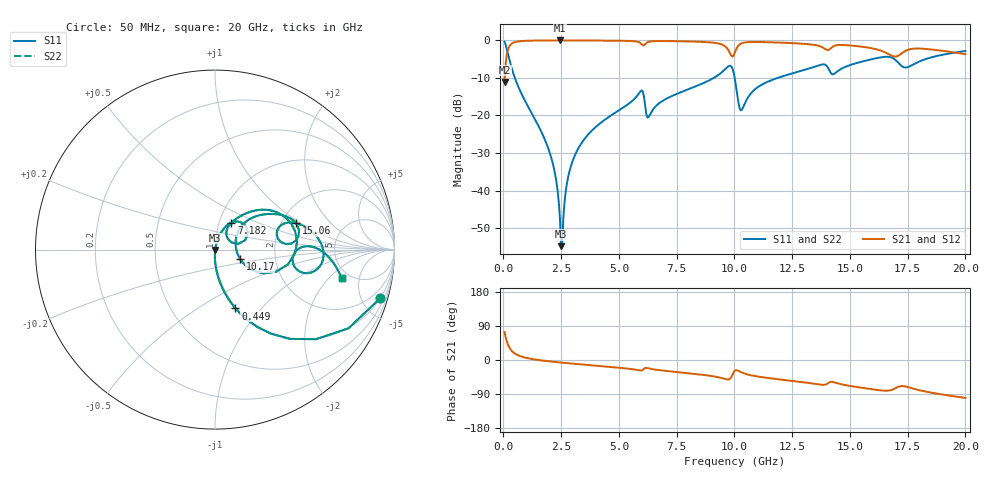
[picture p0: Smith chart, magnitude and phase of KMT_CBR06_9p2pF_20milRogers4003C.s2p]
! Data measured by Modelithics Inc. support@modelithics.com 813-866-6335
! KEMET CBR0603 9.2pF, Pad Width= 0.851mm, Pad Length= 0.64mm, Pad Gap= 0.62mm, 20mil Rogers 4003C substrate Data, January 2022
# hz S ma R 50
! 2 Port Network Data from SP1.SP block
! freq  magS11  angS11  magS21  angS21  magS12  angS12  magS22  angS22
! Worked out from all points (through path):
!   401 points, 50 MHz to 20 GHz, reference 50 ohm
!   highest |S21| = -0.01 dB at 2.444 GHz (marker M1); lowest = -11.1 dB at 50 MHz (marker M2)
!   group delay of S21, straight-line fit = 14.5 ps
!   lowest |S11| = -54.8 dB at 2.494 GHz (marker M3), VSWR 1.00, Z = 50.1 - j0.146 ohm
!   |S11| at or under -10 dB: 495.2 MHz to 9.103 GHz (8.608 GHz wide, 179 % of centre); 10.01 GHz to 11.87 GHz (1.858 GHz wide, 17 % of centre)
!   |S22| runs from -54.8 to -0.4 dB; largest |S21 - S12| = 0
!   S11 on the Smith chart (normalised r, x): 50 MHz: 0.99, -6.81; 449 MHz: 0.99, -0.73; 7.182 GHz: 1.14, +0.35; 10.17 GHz: 1.31, -0.14; 15.06 GHz: 2.41, +0.91; 20 GHz: 4.24, -2.85
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5e7  0.9599 -16.4  0.2798 73.6  0.2798 73.6  0.9599 -16.4
4.49e8  0.3471 -70.8  0.9371 19.1  0.9371 19.1  0.3471 -70.8
1.995125e9  0.03251 -91.6  0.9983 -3.6  0.9983 -3.6  0.03251 -91.6
2.294375e9  0.013 -90.2  0.9986 -5.5  0.9986 -5.5  0.013 -90.2
2.444e9  0.004323 -79.8  0.9987 -6.5  0.9987 -6.5  0.004323 -79.8
2.493875e9  0.001817 -53.3  0.9987 -6.8  0.9987 -6.8  0.001817 -53.3
2.892875e9  0.01975 77.1  0.9984 -9.1  0.9984 -9.1  0.01975 77.1
3.391625e9  0.04341 76.3  0.9975 -11.8  0.9975 -11.8  0.04341 76.3
5.93525e9  0.2104 46.1  0.9209 -27.9  0.9209 -27.9  0.2104 46.1
6.284375e9  0.09528 44.0  0.9574 -22.1  0.9574 -22.1  0.09528 44.0
6.73325e9  0.145 60.0  0.9808 -26.7  0.9808 -26.7  0.145 60.0
7.182125e9  0.1751 58.6  0.9789 -29.7  0.9789 -29.7  0.1751 58.6
9.476375e9  0.3819 34.7  0.8767 -48.0  0.8767 -48.0  0.3819 34.7
9.8255e9  0.4597 5.7  0.6589 -48.6  0.6589 -48.6  0.4597 5.7
1.0025e10  0.3007 -26.1  0.699 -27.7  0.699 -27.7  0.3007 -26.1
1.017462e10  0.1474 -20.2  0.8537 -28.9  0.8537 -28.9  0.1474 -20.2
1.097262e10  0.2339 42.1  0.953 -43.2  0.953 -43.2  0.2339 42.1
1.336662e10  0.435 25.3  0.879 -61.9  0.879 -61.9  0.435 25.3
1.506238e10  0.4757 17.9  0.8538 -69.0  0.8538 -69.0  0.4757 17.9
1.670825e10  0.6016 -6.3  0.6496 -80.4  0.6496 -80.4  0.6016 -6.3
1.74065e10  0.4353 -6.4  0.7253 -69.8  0.7253 -69.8  0.4353 -6.4
2e10  0.7232 -12.8  0.656 -100.0  0.656 -100.0  0.7232 -12.8
